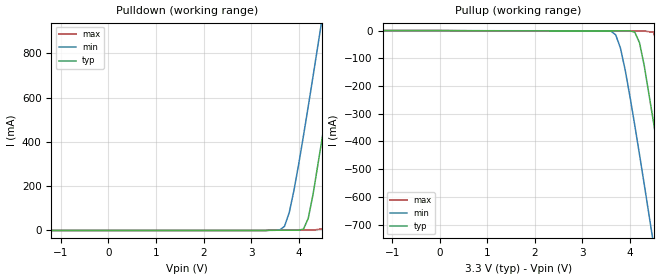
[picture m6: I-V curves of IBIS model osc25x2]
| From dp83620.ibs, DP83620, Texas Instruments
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|   Model osc25x2
[Model]   osc25x2
Model_type   Output
Polarity   Inverting
Enable   Active-High
Vmeas = 1.5000V
C_comp   1.0000pF   1.0000pF   1.0000pF
[Temperature Range]   25.0000   0.1250k   -40.0000
[Voltage Range]   3.3000V   3.0000V   3.6000V
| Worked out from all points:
|   slope of the pullup table from 0 to 0.495 V, typ, clamps not added: 1.19 kohm
[Pulldown]
| voltage   I(typ)   I(min)   I(max)
-3.3V     0A         0A         0A
3.6V      1.099mA    2.318mA    1.555mA
3.7V      1.103mA    18.37mA    1.56mA
3.8V      1.11mA     80.08mA    1.567mA
4.1V      6.217mA    428mA      1.603mA
4.2V      54.57mA    559.8mA    1.639mA
4.5V      425.9mA    967.9mA    7.417mA
4.7V      707.9mA    1.245A     200.5mA
4.9V      996mA      1.525A     486.1mA
5.1V      1.287A     1.806A     783.4mA
5.3V      1.58A      2.089A     1.085A
6.6V      3.503A     3.939A     3.076A
[Pullup]
| voltage   I(typ)   I(min)   I(max)
-3.3V     0A         0A         0A
3.6V      -1.081mA   -2.06mA    -1.527mA
3.7V      -1.083mA   -15.55mA   -1.53mA
3.8V      -1.086mA   -63.14mA   -1.534mA
4.1V      -5.367mA   -340.7mA   -1.543mA
4.2V      -43.48mA   -446.6mA   -1.551mA
4.5V      -335.7mA   -775mA     -6.395mA
4.7V      -559.6mA   -998.5mA   -156mA
4.9V      -788.6mA   -1.224A    -379.2mA
5.1V      -1.02A     -1.451A    -612.3mA
5.3V      -1.253A    -1.678A    -849mA
6.6V      -2.784A    -3.17A     -2.413A
[Ramp]
| variable   typ   min   max
dV/dt_r   1.7737/0.4988n   1.5328/0.7567n   1.9870/0.3615n
dV/dt_f   1.8364/0.4766n   1.5967/0.7630n   2.0404/0.3438n
R_load = 10.0000k
